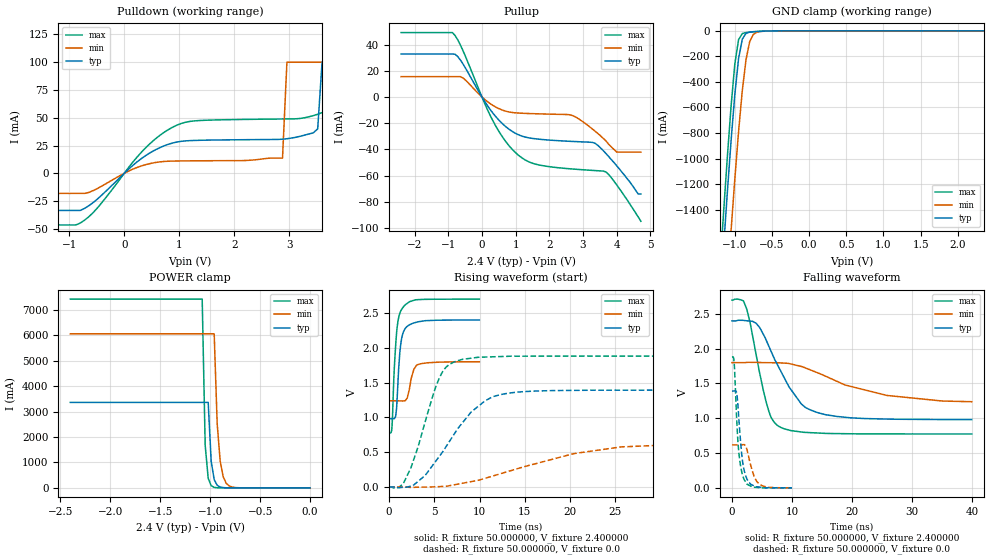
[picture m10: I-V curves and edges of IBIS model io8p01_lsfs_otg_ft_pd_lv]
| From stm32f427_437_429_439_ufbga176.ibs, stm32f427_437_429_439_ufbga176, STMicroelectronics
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|   Model io8p01_lsfs_otg_ft_pd_lv
[Model]  io8p01_lsfs_otg_ft_pd_lv
Model_type I/O
Polarity   Non-Inverting
Enable   Active-Low
Vinl =   0.720000V
Vinh =   1.680000V
Vmeas =  1.200000V
Cref =   50.000000pF
Rref =   100.000000M
Vref =   0.0V
C_comp   7.971100pF   7.737700pF   8.264100pF
[Temperature Range]   25.000000   0.125000k   -40.000000
[Pullup Reference]   2.400000V   1.800000V   2.700000V
[Pulldown Reference]   0.0V   0.0V   0.0V
[POWER Clamp Reference]   2.400000V   1.800000V   2.700000V
[GND Clamp Reference]   0.0V   0.0V   0.0V
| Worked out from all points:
|   slope of the pulldown table from 0 to 0.36 V, typ, clamps not added: 24.1 ohm
|   slope of the pullup table from 0 to 0.36 V, typ, clamps not added: 26.8 ohm
|   GND clamp passes 1 mA (typ) near -0.52 V on its own axis
|   POWER clamp passes 1 mA (typ) near -0.81 V on its own axis
|   rising waveform, R_fixture 50.000000, V_fixture 2.400000: 20-80 % time 480ps typ, 592ps min, 492ps max; typ from 0.981 V to 2.4 V
|   rising waveform, R_fixture 50.000000, V_fixture 0.0: 20-80 % time 4.78ns typ, 10.6ns min, 2.68ns max; typ from 0 V to 1.39 V
|   falling waveform, R_fixture 50.000000, V_fixture 2.400000: 20-80 % time 5.32ns typ, 11.5ns min, 2.78ns max; typ from 2.4 V to 0.981 V
|   falling waveform, R_fixture 50.000000, V_fixture 0.0: 20-80 % time 912ps typ, 1.27ns min, 796ps max; typ from 1.39 V to 0 V
[Pulldown]
|Voltage   I(typ)   I(min)   I(max)
-2.4V     -33.44mA   -18.12mA   -46.52mA
-800mV    -33.44mA   -18.12mA   -44.78mA
1.04V     28.81mA    11.14mA    44.91mA
2.88V     30.7mA     13.64mA    48.89mA
2.96V     31.11mA    100mA      48.94mA
3.52V     40mA       100mA      53.15mA
3.6V      100mA      100mA      54.65mA
3.92V     100mA      100mA      60mA
4V        100mA      100mA      100mA
4.4V      100mA      100mA      100mA
4.48V     100mA      100mA      1A
4.8V      100mA      100mA      1A
[Pullup]
|Voltage   I(typ)   I(min)   I(max)
-2.4V     32.78mA    15.54mA    49.16mA
-880mV    32.78mA    15.54mA    49.16mA
-560mV    25.06mA    14.45mA    35.14mA
320mV     -12.14mA   -6.322mA   -17.91mA
960mV     -27.18mA   -12mA      -41.54mA
1.52V     -31.65mA   -12.71mA   -50.68mA
2.64V     -33.82mA   -13.73mA   -54.81mA
3.36V     -35.34mA   -26.1mA    -56.1mA
3.68V     -43.1mA    -33.4mA    -57.12mA
4V        -52.4mA    -42mA      -67mA
4.64V     -74mA      -42mA      -91.5mA
4.72V     -74mA      -42mA      -94.8mA
[GND_clamp]
|Voltage   I(typ)   I(min)   I(max)
-2.4V     -9.765A    -9.942A    -9.572A
-1.2V     -2.124A    -2.851A    -1.855A
-1.15V    -1.682A    -2.408A    -1.408A
-1.1V     -1.256A    -1.975A    -979.8mA
-1.05V    -854.9mA   -1.557A    -584.5mA
-1V       -496.5mA   -1.158A    -257.5mA
-950mV    -217.7mA   -789.7mA   -69.53mA
-900mV    -65.58mA   -469.8mA   -21.52mA
-850mV    -19.65mA   -226.4mA   -13.58mA
-800mV    -9.766mA   -84.22mA   -10.49mA
-700mV    -4.935mA   -9.894mA   -5.821mA
2.35V     58.09uA    37.92uA    67.25uA
[POWER_clamp]
|Voltage   I(typ)   I(min)   I(max)
-2.4V     3.365A     6.064A     7.43A
-1.08V    3.365A     6.064A     7.43A
-1.05V    3.365A     6.064A     1.669A
-1.02V    3.365A     6.064A     375mA
-990mV    1.047A     6.064A     84.24mA
-960mV    325.6mA    6.064A     18.93mA
-930mV    101.3mA    2.529A     4.252mA
-900mV    31.51mA    1.055A     955.2uA
-870mV    9.804mA    440.1mA    214.6uA
-840mV    3.05mA     183.6mA    74.58uA
-720mV    28.58uA    5.557mA    74.58uA
0V        0A         0A         0A
[Ramp]
| variable   typ   min   max
dV/dt_r  0.83478/4.77807n   0.36949/10.63421n   1.12806/2.67656n
dV/dt_f  0.85112/5.31517n   0.32622/11.65562n   1.15474/2.78165n
R_load = 50.000000
[Rising Waveform]
R_fixture= 50.000000
V_fixture= 2.400000
V_fixture_min= 1.800000
V_fixture_max= 2.700000
|time   V(typ)   V(min)   V(max)
0s        980.6mV    1.238V     774.4mV
300.3ps   980.3mV    1.238V     836.8mV
520.5ps   981.6mV    1.238V     1.574V
720.7ps   1.021V     1.238V     2.038V
900.9ps   1.321V     1.238V     2.313V
1.161ns   1.902V     1.237V     2.487V
1.401ns   2.148V     1.236V     2.557V
2.002ns   2.309V     1.281V     2.639V
3.043ns   2.368V     1.751V     2.69V
9.97ns    2.399V     1.799V     2.699V
[Rising Waveform]
R_fixture= 50.000000
V_fixture= 0.0
V_fixture_min= 0.0
V_fixture_max= 0.0
|time   V(typ)   V(min)   V(max)
0s        15.26uV    8.526uV    105.5uV
1.602ns   -4.898mV   44.11uV    59.16mV
3.203ns   81.37mV    -2.585mV   580.7mV
5.365ns   408.5mV    4.265mV    1.51V
6.166ns   555.4mV    8.755mV    1.703V
7.207ns   763.3mV    31.74mV    1.798V
10.57ns   1.235V     123.3mV    1.867V
13.21ns   1.348V     225.6mV    1.878V
25.63ns   1.391V     575.7mV    1.88V
39.88ns   1.391V     617.3mV    1.88V
[Falling Waveform]
R_fixture= 50.000000
V_fixture= 2.400000
V_fixture_min= 1.800000
V_fixture_max= 2.700000
|time   V(typ)   V(min)   V(max)
0s        2.399V     1.799V     2.699V
2.402ns   2.401V     1.802V     2.582V
4.004ns   2.365V     1.803V     1.92V
5.686ns   2.123V     1.799V     1.233V
6.567ns   1.95V      1.798V     1.004V
7.848ns   1.722V     1.796V     881.1mV
11.53ns   1.206V     1.744V     802.7mV
14.81ns   1.068V     1.634V     785.9mV
25.79ns   988.5mV    1.328V     774.8mV
39.88ns   980.6mV    1.238V     774.4mV
[Falling Waveform]
R_fixture= 50.000000
V_fixture= 0.0
V_fixture_min= 0.0
V_fixture_max= 0.0
|time   V(typ)   V(min)   V(max)
0s        1.391V     617.3mV    1.88V
360.4ps   1.392V     617.3mV    1.802V
840.8ps   1.329V     617.2mV    887.7mV
1.281ns   830.2mV    616.8mV    403.7mV
1.642ns   463.5mV    618.7mV    223.4mV
2.002ns   262.1mV    621.2mV    122.6mV
2.743ns   88.15mV    459.3mV    42.09mV
3.684ns   27.4mV     165.3mV    8.772mV
4.484ns   11.97mV    57.43mV    4.017mV
9.97ns    15.26uV    8.526uV    105.5uV
